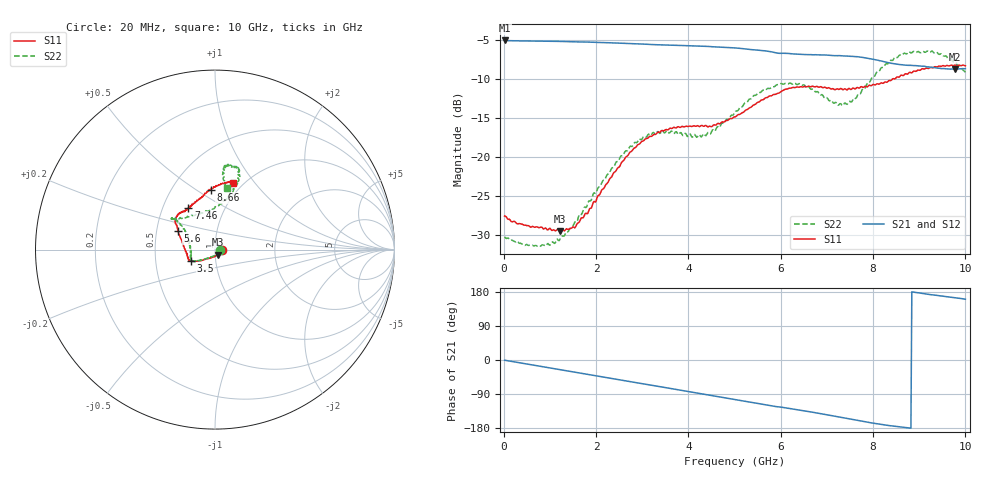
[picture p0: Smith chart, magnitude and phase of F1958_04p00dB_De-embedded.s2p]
! Integrated Device Technology
! Corporate Headquarters
! 6024 Silver Creek Valley Road
! San Jose, CA 95138  USA
! Phone:  1-408-284-8200
! Toll Free:  1-800-223-1366
! Webpage:  http://www.idt.com/
! Timing and RF Division
! 515 Groton Road, Suite 102
! Westford, MA 01886-6024
! Device:  F1958
! Description: 7-bit 0.25 dB Digital Step Attenuator
! Frequency:  0.001 -  6.000 GHz
! Package:  4x4 mm Thin QFN Plastic Package: 24 pin
! Ports:  2 RF, 12 DC
!  Pin  1  = D0
!  Pin  2  = VDD
!  Pin  3  = VMODE
!  Pin  4  = GND
!  Pin  5  = RF1  =  Port 1
!  Pin  6  = GND
!  Pin  7  = GND
!  Pin  8  = GND
!  Pin  9  = GND
!  Pin 10  = GND
!  Pin 11  = GND
!  Pin 12  = GND
!  Pin 13  = GND
!  Pin 14  = RF2  =  Port 2
!  Pin 15  = GND
!  Pin 16  = LE
!  Pin 17  = CLK
!  Pin 18  = DATA
!  Pin 19  = D6
!  Pin 20  = D5
!  Pin 21  = D4
!  Pin 22  = D3
!  Pin 23  = D2
!  Pin 24  = D1
! State:  16
! Atten State:  4.00 dB
! Voltage:  +3.30 Volts
! Current:  0.258 mA
! Data:  The device was measured on a F1958 evaluation board which has
!  individual transmission lines to the RF pins.  Data was collected
!  using a calibrated network analyzer.  The evaluation board was
!  de-embedded using Automatic Fixture Removal (AFR).
!  The reference plane is the edge of the package pin.
! Misc:
!  Action Tracker AT0419
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# GHz S dB R 50
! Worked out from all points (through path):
!   500 points, 20 MHz to 10 GHz, reference 50 ohm
!   highest |S21| = -5.01 dB at 20 MHz (marker M1); lowest = -8.7 dB at 9.78 GHz (marker M2)
!   group delay of S21, straight-line fit = 56.5 ps
!   lowest |S11| = -29.5 dB at 1.22 GHz (marker M3), VSWR 1.07, Z = 51.7 - j2.92 ohm
!   |S11| at or under -10 dB: start of sweep to 8.416 GHz
!   |S22| runs from -31.5 to -6.4 dB; largest |S21 - S12| = 0.0014
!   S11 on the Smith chart (normalised r, x): 20 MHz: 1.09, -0.00; 3.5 GHz: 0.76, -0.10; 5.6 GHz: 0.64, +0.14; 7.46 GHz: 0.68, +0.34; 8.66 GHz: 0.77, +0.57; 10 GHz: 0.90, +0.79
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0.02  -27.60 -3.0  -5.01 -0.6  -5.01 -0.5  -30.28 -3.8
0.76  -29.10 -26.1  -5.09 -15.9  -5.09 -15.9  -31.39 -37.4
1.22  -29.53 -57.8  -5.13 -25.5  -5.13 -25.5  -30.58 -77.8
1.52  -29.04 -83.0  -5.18 -31.8  -5.17 -31.7  -28.65 -103.1
1.7  -27.81 -96.6  -5.20 -35.4  -5.20 -35.4  -27.26 -114.9
2.64  -20.04 -141.8  -5.39 -55.0  -5.37 -55.0  -19.23 -145.2
2.98  -18.06 -148.9  -5.47 -62.1  -5.46 -62.2  -17.80 -149.4
3.36  -16.82 -153.1  -5.57 -69.9  -5.57 -70.0  -16.85 -153.1
3.5  -16.50 -155.1  -5.59 -72.7  -5.60 -72.9  -16.86 -156.9
4.32  -16.04 -167.3  -5.75 -89.7  -5.76 -89.7  -17.06 175.8
5.02  -14.84 170.0  -5.98 -104.5  -5.99 -104.5  -14.14 148.5
5.6  -12.65 153.3  -6.32 -116.7  -6.33 -116.7  -11.48 142.5
6.16  -11.20 143.4  -6.68 -127.5  -6.70 -127.4  -10.61 144.2
6.68  -10.91 135.8  -6.85 -137.6  -6.86 -137.5  -11.28 139.9
7.22  -11.23 128.0  -6.97 -149.1  -6.98 -148.9  -13.19 116.6
7.46  -11.25 122.6  -7.02 -154.4  -7.03 -154.3  -13.06 97.1
7.94  -10.81 112.3  -7.36 -165.4  -7.36 -165.4  -10.25 75.0
8.34  -10.18 102.1  -7.87 -172.9  -7.88 -173.0  -7.89 71.0
8.66  -9.51 94.2  -8.17 -177.6  -8.17 -177.5  -6.70 72.9
9.3  -8.51 80.7  -8.47 171.6  -8.49 171.6  -6.48 83.0
9.78  -8.17 76.1  -8.70 164.3  -8.73 164.3  -7.79 83.1
10  -8.27 74.9  -8.63 160.3  -8.66 160.4  -9.11 79.2
